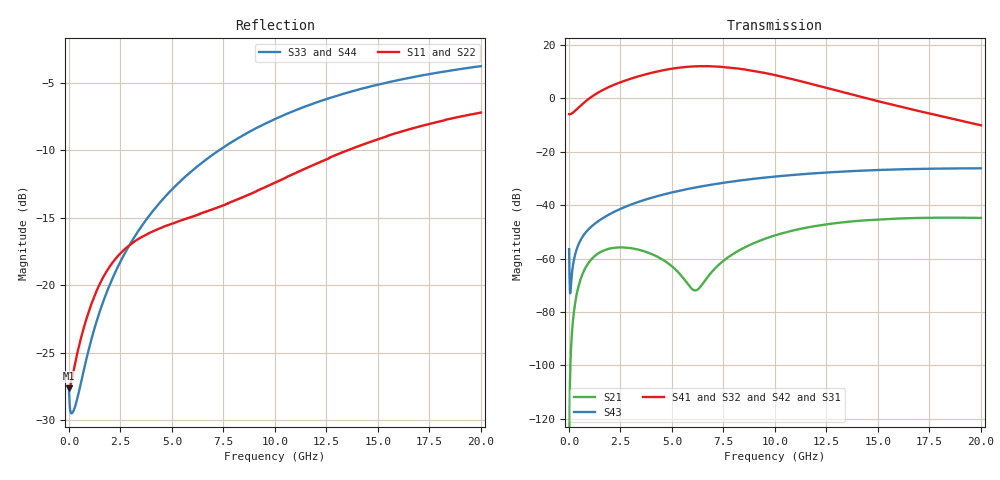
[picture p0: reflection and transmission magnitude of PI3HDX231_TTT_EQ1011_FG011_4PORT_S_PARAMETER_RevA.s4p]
! NPort=4 DATA=2000 NOISE=0 GROUPDELAY=0 COMPLEX_DATAFORMAT=POLAR
! NumOfBlock=1 NumOfParam=0
! .MODEL Smodel S TSTONEFILE=PI3HDX231_TTT_EQ1011_FG011_4PORT_S_PARAMETER_RevA.s4p TYPE=S
!  -- The above .MODEL line can be used for the S element in the netlist.
! The s parameter is extracted from the linear redriver, it is not bi-directional; only s(4,1)s(4,2) and s(3,1)s(3,2)
! should be the insertion loss
!Port definition:
!Port1 = input+
!Port2 = input-
!Port3 = output+
!Port4 = output-
# Hz S MA R  50
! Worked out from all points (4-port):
!   2000 points, 10 MHz to 20 GHz, reference 50 ohm
!   strongest paths, dB at 10 MHz, 5.01 GHz, 10.01 GHz, 15.01 GHz, 20 GHz:
!     S41: -5.9, 11.1, 8.7, -1.1, -10.1
!     S32: -5.9, 11.1, 8.7, -1.0, -10.0
!     S42: -5.9, 11.1, 8.6, -1.3, -10.2
!     S31: -5.9, 11.0, 8.5, -1.4, -10.5
!     S43: -56.5, -35.2, -29.3, -26.9, -26.2
!     S21: -134.8, -63.0, -51.3, -45.4, -44.8
!   lowest |S11| = -27.6 dB at 10 MHz (marker M1), VSWR 1.09, Z = 46 - j0.0776 ohm
!   |S11| at or under -10 dB: start of sweep to 13.55 GHz
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1e7  0.04152 -178.8  1.825e-07 -14.0  0 0.0  0 0.0
     1.825e-07 -13.9  0.04152 -178.8  0 0.0  0 0.0
     0.5042 0.1  0.5042 -179.9  0.04012 -3.2  0.0015 -70.3
     0.5042 -179.9  0.5042 0.1  0.0015 -70.3  0.04012 -3.2
4.08e9  0.1584 -140.9  0.001185 -4.5  1.841e-10 -144.9  1.261e-10 -129.7
        0.001185 -4.4  0.1585 -141.0  1.224e-10 -130.0  1.903e-10 -144.4
        3.023 -41.7  3.029 138.1  0.1884 -99.5  0.01401 66.3
        3.047 138.1  3.04 -41.0  0.01399 66.2  0.1884 -99.5
6.01e9  0.1797 -138.2  0.0002579 26.8  1.912e-09 152.9  1.132e-09 -171.6
        0.000263 27.4  0.1795 -138.4  1.095e-09 -171.0  1.99e-09 152.5
        3.908 -102.5  3.925 77.3  0.2665 -105.4  0.021 55.8
        3.95 77.1  3.94 -101.8  0.02093 55.8  0.2666 -105.4
8.02e9  0.2051 -133.4  0.001253 100.7  9.784e-09 91.2  6.792e-09 136.9
        0.001252 100.2  0.2045 -133.7  6.614e-09 138.3  1.017e-08 90.0
        3.63 -168.1  3.668 11.7  0.3428 -110.7  0.02808 43.4
        3.688 11.3  3.666 -167.2  0.02797 43.5  0.343 -110.8
1.06e10  0.2521 -128.9  0.003159 78.6  3.919e-08 21.4  3.155e-08 61.8
         0.003152 78.3  0.2507 -129.0  3.117e-08 63.7  4.019e-08 19.4
         2.352 117.9  2.407 -62.5  0.4313 -117.1  0.03611 26.6
         2.413 -63.1  2.382 119.0  0.03599 26.8  0.4314 -117.1
1.361e10  0.3174 -128.4  0.004921 47.3  1.114e-07 -46.9  9.03e-08 -16.3
          0.004904 47.1  0.3154 -128.4  9.057e-08 -14.5  1.125e-07 -49.0
          1.166 52.1  1.214 -129.3  0.5179 -123.7  0.0432 7.0
          1.21 -130.0  1.186 53.4  0.04312 7.2  0.5178 -123.8
2e10  0.4355 -135.6  0.00579 -4.1  3.705e-07 -160.9  2.771e-07 -141.2
      0.005761 -4.2  0.4338 -135.4  2.818e-07 -140.2  3.679e-07 -162.5
      0.2995 -48.1  0.3166 126.7  0.6464 -135.0  0.04883 -32.3
      0.3127 126.3  0.3084 -46.8  0.04893 -32.1  0.6461 -135.0
